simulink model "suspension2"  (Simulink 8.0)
settings: Solver=ode45  StartTime=0.0  StopTime=10.0  RelTol=1e-3
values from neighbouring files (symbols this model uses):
  a11y = a{1,:}    [suspension_2.m]    (also in suspension_3.m)
  a11z = a{1,:}    [suspension_2.m]    (also in suspension_3.m)
  b11y = b{1,:}    [suspension_2.m]    (also in suspension_3.m)
  b11z = b{1,:}    [suspension_2.m]    (also in suspension_3.m)
  b12y = b{2,:}    [suspension_2.m]    (also in suspension_3.m)
  b12z = b{2,:}    [suspension_2.m]    (also in suspension_3.m)
  b13y = b{3,:}    [suspension_2.m]    (also in suspension_3.m)
  b13z = b{3,:}    [suspension_2.m]    (also in suspension_3.m)
  b14y = b{4,:}    [suspension_2.m]    (also in suspension_3.m)
  b14z = b{4,:}    [suspension_2.m]    (also in suspension_3.m)
  C = [c -c;-c ct+c]    [rad_aufhaeng_1.m]    (also in rad_aufhaeng_2.m; rad_aufhaeng_3.m; rad_aufhaeng_4.m; suspension_1.m = [c*(a^2 + (L-a)^2) c*L -c*a c*(L-a))
  delay = (L/v)    (= 0.1)    [suspension_2.m]    (also in suspension_3.m)
  dt = 0.001    [coulomb_1.m]    (also in coulomb_10.m; coulomb_11.m; coulomb_2.m; coulomb_3.m)
  K = [k -k; -k kt+k]    [rad_aufhaeng_1.m]    (also in rad_aufhaeng_2.m; rad_aufhaeng_3.m; rad_aufhaeng_4.m; suspension_1.m = [k*(a^2+(L-a)^2) k*L -k*a k*(L-a))
  M = [ms 0;0 ma]    [rad_aufhaeng_1.m]    (also in rad_aufhaeng_2.m; rad_aufhaeng_3.m; rad_aufhaeng_4.m; suspension_1.m = [I 0 0 0;0 ms 0 0;0 0 ma 0;0 0 0 ma])
  varianz = 1e-6    (= 1e-06)    [diff_filter_1.m]    (also in diff_filter_2.m = 1e-08; rad_aufhaeng_4.m = 2e-06; suspension_2.m = 2e-06; suspension_3.m = 2e-06)
  x0v0 = [0 0.002 0 0 0.01 0 0 0]'    [suspension_2.m]    (also in suspension_3.m)

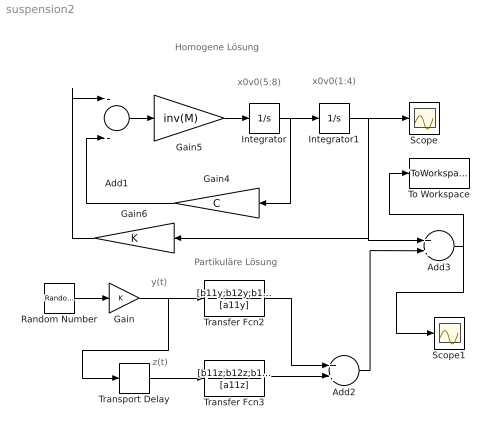
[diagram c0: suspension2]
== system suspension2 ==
  note: z(t)
  note: y(t)
  note: Partikuläre Lösung
  note: Homogene Lösung
  note: x0v0(1:4)
  note: x0v0(5:8)
  Add1 : Sum  Inputs=--
  Add2 : Sum
  Add3 : Sum
  Gain : Gain
  Gain4 : Gain  Gain=C  Multiplication=Matrix(K*u)
  Gain5 : Gain  Gain=inv(M)  Multiplication=Matrix(K*u)
  Gain6 : Gain  Gain=K  Multiplication=Matrix(K*u)
  Integrator : Integrator  InitialCondition=x0v0(5:8, 1)
  Integrator1 : Integrator  InitialCondition=x0v0(1:4,1)
  Random Number : RandomNumber  Variance=varianz  Seed=1395  SampleTime=dt
  Scope : Scope
  Scope1 : Scope
  To Workspace : ToWorkspace  VariableName=y  SampleTime=-1  SaveFormat=Structure With Time
  Transfer Fcn2 : TransferFcn  Numerator=[b11y;b12y;b13y;b14y]  Denominator=[a11y]
  Transfer Fcn3 : TransferFcn  Numerator=[b11z;b12z;b13z;b14z]  Denominator=[a11z]
  Transport Delay : TransportDelay  DelayTime=delay
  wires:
  Add1/1 -> Gain5/1
  Integrator/1 -> Gain4/1, Integrator1/1
  Gain4/1 -> Add1/2
  Gain5/1 -> Integrator/1
  Transfer Fcn2/1 -> Add2/1
  Transfer Fcn3/1 -> Add2/2
  Gain6/1 -> Add1/1
  Add2/1 -> Add3/2
  Integrator1/1 -> Scope/1, Add3/1, Gain6/1
  Transport Delay/1 -> Transfer Fcn3/1
  Random Number/1 -> Gain/1
  Add3/1 -> Scope1/1, To Workspace/1
  Gain/1 -> Transport Delay/1, Transfer Fcn2/1
